| TEXAS INSTRUMENTS INCORPORATED
| Standard Linear and Logic Group
| IBIS Model of SN74CB3T16211
| 3.3-V LOW-VOLTAGE 14-BIT FET BUS SWITCH WITH 5-V-TOLERANT/LEVEL SHIFTER
| This file contains package information for the following:
|  VFBGA 56-pin (GQL) package as [Component] CB3T16211_GQL
|  TSSOP 56-pin (DGG) package as [Component] CB3T16211_DGG
|  TVSOP 56-pin (DGV) package as [Component] CB3T16211_DGV
|  SSOP 56-pin (DL) package as [Component] CB3T16211_DL
| This device can be powered at the following Vccs:
|  3.3 volt Vcc
|  2.5 volt Vcc
| This file provides unique models under the [Model Selector] for each Vcc.
| For operation at a specific Vcc, select the appropriate model after each
| [Model Selector] keyword.
[IBIS Ver]   3.2
[Comment char]  |_char
[File Name]   sn74cb3t16211.ibs
[File Rev]   1.3 | a_die
[Date]   March 23, 2006
[Source]   Data created from TI-SPICE simulations at TI-SLL.
[Notes]   The following is an IBIS list for the CB3T16211.
   Please contact sllibis@ti.com with questions and
   comments concerning SLL IBIS models.
   - FILE REV HISTORY
   - 1.3 Added GQL package information on 03/23/06
   - Non-monotonic data due to FET characteristics.
   - Power clamp data deleted as there is no power-clamp diode.
[Disclaimer] Property of Texas Instruments Incorporated.  Unauthorized
   reproduction and/or distribution is strictly prohibited.
   This product is protected under copyright law.
   Created  2003, (C) Copyright  2003, Texas Instruments
   Incorporated, All Rights Reserved
   UNLESS THERE IS A SIGNED, WRITTEN AGREEMENT TO THE
   CONTRARY, TEXAS INSTRUMENTS (TI) IS PROVIDING THE IBIS
   MODELS  AND WITHOUT ANY WARRANTY, EXPRESSED OR
   IMPLIED.  TI assumes no liability for:
   1) the accuracy of the IBIS models provided to your
   company;
   2) the proper functioning of these IBIS Models in your
   design or for any resulting applications; or
   3) infringement of patents, copyrights or intellectual
   property rights resulting from your use of these IBIS
   models.
   TI provides IBIS Models as a service to our customers.
   You and your company shall not distribute, sell or give
   these models to anyone else without prior written
   permission from TI.
   TI reserves the right to make changes to our products or
   to discontinue any semiconductor product or service
   without notice, and advises our customers to obtain the
   latest version of relevant information to verify, before
   placing orders, that the information being relied on is
   current.
   Please be aware that your receipt and use of the IBIS
   information provided shall serve as acceptance of these
   terms and conditions.  If you do not accept these terms,
   you should return or destroy the IBIS models and any
   other accompanying information immediately.
| Component CB3T16211_GQL 56-pin VFBGA
[Component]   CB3T16211_GQL
[Manufacturer]   Texas Instruments, Inc.
[Package]
|   typ   min   max
R_pkg   6.500e-02   3.500e-02   9.700e-02
L_pkg   1.952e-09   1.000e-09   3.191e-09
C_pkg   2.830e-13   1.620e-13   4.340e-13
[Pin]   signal_name   model_name   R_pin   L_pin   C_pin
A3   NC   NC   3.600e-02   1.004e-09   1.760e-13
A2   1A1   CB3T16211_IO   4.000e-02   1.191e-09   1.860e-13
A1   1A2   CB3T16211_IO   4.700e-02   1.411e-09   2.090e-13
B3   1A3   CB3T16211_IO   9.700e-02   3.191e-09   4.340e-13
B2   1A4   CB3T16211_IO   7.400e-02   2.213e-09   3.290e-13
B1   1A5   CB3T16211_IO   6.000e-02   1.712e-09   2.430e-13
C3   1A6   CB3T16211_IO   8.500e-02   2.691e-09   3.680e-13
C2   GND   GND   7.400e-02   2.160e-09   3.150e-13
C1   1A7   CB3T16211_IO   6.000e-02   1.666e-09   2.470e-13
D2   1A8   CB3T16211_IO   7.400e-02   2.121e-09   3.130e-13
D3   1A9   CB3T16211_IO   9.100e-02   2.924e-09   3.970e-13
D1   1A10   CB3T16211_IO   6.000e-02   1.619e-09   2.450e-13
E2   1A11   CB3T16211_IO   6.900e-02   2.031e-09   2.880e-13
E1   1A12   CB3T16211_IO   6.000e-02   1.583e-09   2.200e-13
F1   2A1   CB3T16211_IO   6.000e-02   1.578e-09   2.200e-13
F2   2A2   CB3T16211_IO   6.900e-02   2.017e-09   2.860e-13
G1   VCC   POWER   6.000e-02   1.594e-09   2.410e-13
G3   2A3   CB3T16211_IO   9.200e-02   2.917e-09   3.970e-13
G2   GND   GND   7.500e-02   2.114e-09   3.150e-13
H1   2A4   CB3T16211_IO   6.000e-02   1.632e-09   2.470e-13
H2   2A5   CB3T16211_IO   7.000e-02   2.074e-09   3.070e-13
H3   2A6   CB3T16211_IO   8.600e-02   2.664e-09   3.650e-13
J1   2A7   CB3T16211_IO   6.000e-02   1.689e-09   2.490e-13
J2   2A8   CB3T16211_IO   6.600e-02   2.152e-09   3.320e-13
J3   2A9   CB3T16211_IO   8.700e-02   3.118e-09   4.230e-13
K1   2A10   CB3T16211_IO   3.800e-02   1.303e-09   2.000e-13
K2   2A11   CB3T16211_IO   3.500e-02   1.176e-09   1.830e-13
K3   2A12   CB3T16211_IO   3.500e-02   1.007e-09   1.620e-13
K4   2B12   CB3T16211_IO   3.500e-02   1.000e-09   1.620e-13
K5   2B11   CB3T16211_IO   3.500e-02   1.154e-09   1.800e-13
K6   2B10   CB3T16211_IO   4.100e-02   1.352e-09   2.040e-13
J4   2B9   CB3T16211_IO   8.800e-02   3.137e-09   4.300e-13
J5   2B8   CB3T16211_IO   7.400e-02   2.218e-09   3.340e-13
J6   2B7   CB3T16211_IO   6.000e-02   1.683e-09   2.500e-13
H4   2B6   CB3T16211_IO   8.500e-02   2.658e-09   3.720e-13
H5   2B5   CB3T16211_IO   7.500e-02   2.149e-09   3.210e-13
H6   2B4   CB3T16211_IO   6.000e-02   1.627e-09   2.480e-13
G5   GND   GND   7.500e-02   2.113e-09   3.140e-13
G4   2B3   CB3T16211_IO   9.200e-02   2.922e-09   3.960e-13
G6   2B2   CB3T16211_IO   6.000e-02   1.594e-09   2.420e-13
F5   2B1   CB3T16211_IO   6.900e-02   2.016e-09   2.880e-13
F6   1B12   CB3T16211_IO   6.000e-02   1.580e-09   2.210e-13
E6   1B11   CB3T16211_IO   6.000e-02   1.582e-09   2.200e-13
E5   1B10   CB3T16211_IO   6.900e-02   2.026e-09   2.890e-13
D6   1B9   CB3T16211_IO   6.000e-02   1.610e-09   2.450e-13
D4   1B8   CB3T16211_IO   9.200e-02   2.933e-09   3.960e-13
D5   1B7   CB3T16211_IO   7.500e-02   2.126e-09   3.110e-13
C6   1B6   CB3T16211_IO   6.000e-02   1.641e-09   2.450e-13
C5   GND   GND   7.300e-02   2.168e-09   3.190e-13
C4   1B5   CB3T16211_IO   8.600e-02   2.675e-09   3.620e-13
B6   1B4   CB3T16211_IO   6.000e-02   1.688e-09   2.430e-13
B5   1B3   CB3T16211_IO   7.500e-02   2.281e-09   3.330e-13
B4   1B2   CB3T16211_IO   9.500e-02   3.168e-09   4.240e-12
A6   1B1   CB3T16211_IO   4.500e-02   1.418e-09   2.090e-12
A5   NOE2   CB3T16211_IN   3.900e-02   1.216e-09   1.900e-12
A4   NOE1   CB3T16211_IN   3.700e-02   1.029e-09   1.790e-12
| Component CB3T16211_DGG 56-pin TSSOP
[Component]   CB3T16211_DGG
[Manufacturer]   Texas Instruments, Inc.
[Package]
|   typ   min   max
R_pkg   4.500e-02   3.500e-02   6.200e-02
L_pkg   3.324e-09   2.403e-09   5.094e-09
C_pkg   5.640e-13   3.410e-13   9.140e-13
[Pin]   signal_name   model_name   R_pin   L_pin   C_pin
1   NC   NC   6.200e-02   5.094e-09   8.560e-13
2   1A1   CB3T16211_IO   6.100e-02   4.621e-09   9.020e-13
3   1A2   CB3T16211_IO   6.000e-02   4.316e-09   8.020e-13
4   1A3   CB3T16211_IO   5.900e-02   3.968e-09   6.980e-13
5   1A4   CB3T16211_IO   5.700e-02   3.716e-09   6.490e-13
6   1A5   CB3T16211_IO   4.200e-02   3.517e-09   6.530e-13
7   1A6   CB3T16211_IO   4.100e-02   3.160e-09   5.700e-13
8   GND   GND   3.900e-02   2.981e-09   4.820e-13
9   1A7   CB3T16211_IO   3.900e-02   2.808e-09   4.470e-13
10   1A8   CB3T16211_IO   3.800e-02   2.715e-09   4.090e-13
11   1A9   CB3T16211_IO   4.100e-02   2.675e-09   3.910e-13
12   1A10   CB3T16211_IO   3.900e-02   2.536e-09   3.660e-13
13   1A11   CB3T16211_IO   3.900e-02   2.457e-09   3.480e-13
14   1A12   CB3T16211_IO   3.800e-02   2.411e-09   3.530e-13
15   2A1   CB3T16211_IO   3.900e-02   2.456e-09   3.550e-13
16   2A2   CB3T16211_IO   3.900e-02   2.471e-09   3.490e-13
17   VCC   POWER   4.000e-02   2.580e-09   3.700e-13
18   2A3   CB3T16211_IO   3.800e-02   2.651e-09   3.890e-13
19   GND   GND   3.800e-02   2.739e-09   4.110e-13
20   2A4   CB3T16211_IO   3.900e-02   2.838e-09   4.490e-13
21   2A5   CB3T16211_IO   3.800e-02   2.988e-09   4.840e-13
22   2A6   CB3T16211_IO   3.800e-02   3.104e-09   5.640e-13
23   2A7   CB3T16211_IO   4.000e-02   3.427e-09   6.380e-13
24   2A8   CB3T16211_IO   5.600e-02   3.654e-09   6.410e-13
25   2A9   CB3T16211_IO   5.700e-02   3.932e-09   7.000e-13
26   2A10   CB3T16211_IO   5.800e-02   4.257e-09   8.060e-13
27   2A11   CB3T16211_IO   5.700e-02   4.580e-09   9.140e-13
28   2A12   CB3T16211_IO   5.900e-02   5.038e-09   8.610e-13
29   2B12   CB3T16211_IO   6.000e-02   5.058e-09   8.580e-13
30   2B11   CB3T16211_IO   5.600e-02   4.543e-09   9.040e-13
31   2B10   CB3T16211_IO   5.700e-02   4.241e-09   8.020e-13
32   2B9   CB3T16211_IO   5.900e-02   3.933e-09   6.990e-13
33   2B8   CB3T16211_IO   5.600e-02   3.616e-09   6.370e-13
34   2B7   CB3T16211_IO   3.700e-02   3.368e-09   6.400e-13
35   2B6   CB3T16211_IO   3.600e-02   3.024e-09   5.630e-13
36   2B5   CB3T16211_IO   3.500e-02   2.876e-09   4.740e-13
37   2B4   CB3T16211_IO   3.500e-02   2.745e-09   4.440e-13
38   GND   GND   3.700e-02   2.683e-09   4.050e-13
39   2B3   CB3T16211_IO   3.800e-02   2.603e-09   3.820e-13
40   2B2   CB3T16211_IO   3.800e-02   2.510e-09   3.620e-13
41   2B1   CB3T16211_IO   3.600e-02   2.412e-09   3.410e-13
42   1B12   CB3T16211_IO   3.800e-02   2.416e-09   3.490e-13
43   1B11   CB3T16211_IO   3.800e-02   2.403e-09   3.490e-13
44   1B10   CB3T16211_IO   3.700e-02   2.429e-09   3.410e-13
45   1B9   CB3T16211_IO   3.600e-02   2.483e-09   3.580e-13
46   1B8   CB3T16211_IO   3.700e-02   2.614e-09   3.810e-13
47   1B7   CB3T16211_IO   3.500e-02   2.669e-09   4.020e-13
48   1B6   CB3T16211_IO   3.600e-02   2.763e-09   4.420e-13
49   GND   GND   3.600e-02   2.942e-09   4.780e-13
50   1B5   CB3T16211_IO   3.500e-02   3.053e-09   5.640e-13
51   1B4   CB3T16211_IO   3.600e-02   3.408e-09   6.410e-13
52   1B3   CB3T16211_IO   5.800e-02   3.698e-09   6.410e-13
53   1B2   CB3T16211_IO   5.900e-02   3.974e-09   6.970e-13
54   1B1   CB3T16211_IO   6.100e-02   4.327e-09   8.020e-13
55   NOE2   CB3T16211_IN   6.100e-02   4.624e-09   9.050e-13
56   NOE1   CB3T16211_IN   6.000e-02   5.063e-09   8.580e-13
| Component CB3T16211_DGV 56-pin TVSOP
[Component]   CB3T16211_DGV
[Manufacturer]   Texas Instruments, Inc.
[Package]
|   typ   min   max
R_pkg   6.300e-02   5.000e-02   8.400e-02
L_pkg   2.945e-09   2.394e-09   3.939e-09
C_pkg   3.910e-13   2.710e-13   5.880e-13
[Pin]   signal_name   model_name   R_pin   L_pin   C_pin
1   NC   NC   6.800e-02   3.933e-09   5.880e-13
2   1A1   CB3T16211_IO   6.800e-02   3.568e-09   5.870e-13
3   1A2   CB3T16211_IO   7.600e-02   3.464e-09   5.150e-13
4   1A3   CB3T16211_IO   8.400e-02   3.444e-09   4.590e-13
5   1A4   CB3T16211_IO   8.100e-02   3.277e-09   4.270e-13
6   1A5   CB3T16211_IO   7.400e-02   3.136e-09   3.870e-13
7   1A6   CB3T16211_IO   6.900e-02   2.970e-09   4.010e-13
8   GND   GND   5.000e-02   2.785e-09   3.790e-13
9   1A7   CB3T16211_IO   5.100e-02   2.685e-09   3.200e-13
10   1A8   CB3T16211_IO   5.300e-02   2.611e-09   3.160e-13
11   1A9   CB3T16211_IO   5.300e-02   2.495e-09   2.970e-13
12   1A10   CB3T16211_IO   5.300e-02   2.435e-09   2.920e-13
13   1A11   CB3T16211_IO   5.500e-02   2.412e-09   2.850e-13
14   1A12   CB3T16211_IO   5.600e-02   2.401e-09   2.730e-13
15   2A1   CB3T16211_IO   5.500e-02   2.401e-09   2.730e-13
16   2A2   CB3T16211_IO   5.500e-02   2.399e-09   2.840e-13
17   VCC   POWER   5.400e-02   2.406e-09   2.890e-13
18   2A3   CB3T16211_IO   5.300e-02   2.450e-09   2.930e-13
19   GND   GND   5.100e-02   2.544e-09   3.110e-13
20   2A4   CB3T16211_IO   5.100e-02   2.626e-09   3.150e-13
21   2A5   CB3T16211_IO   5.000e-02   2.727e-09   3.690e-13
22   2A6   CB3T16211_IO   6.500e-02   2.903e-09   3.930e-13
23   2A7   CB3T16211_IO   7.500e-02   3.091e-09   3.860e-13
24   2A8   CB3T16211_IO   8.200e-02   3.272e-09   4.280e-13
25   2A9   CB3T16211_IO   8.200e-02   3.393e-09   4.570e-13
26   2A10   CB3T16211_IO   7.300e-02   3.380e-09   5.080e-13
27   2A11   CB3T16211_IO   7.100e-02   3.577e-09   5.800e-13
28   2A12   CB3T16211_IO   6.800e-02   3.937e-09   5.740e-13
29   2B12   CB3T16211_IO   6.900e-02   3.923e-09   5.690e-13
30   2B11   CB3T16211_IO   6.400e-02   3.536e-09   5.740e-13
31   2B10   CB3T16211_IO   7.600e-02   3.428e-09   5.170e-13
32   2B9   CB3T16211_IO   8.100e-02   3.395e-09   4.680e-13
33   2B8   CB3T16211_IO   8.000e-02   3.255e-09   4.310e-13
34   2B7   CB3T16211_IO   7.100e-02   3.064e-09   3.860e-13
35   2B6   CB3T16211_IO   6.100e-02   2.878e-09   3.890e-13
36   2B5   CB3T16211_IO   5.000e-02   2.710e-09   3.630e-13
37   2B4   CB3T16211_IO   5.000e-02   2.606e-09   3.110e-13
38   GND   GND   5.200e-02   2.534e-09   3.060e-13
39   2B3   CB3T16211_IO   5.200e-02   2.439e-09   2.890e-13
40   2B2   CB3T16211_IO   5.300e-02   2.399e-09   2.860e-13
41   2B1   CB3T16211_IO   5.500e-02   2.394e-09   2.820e-13
42   1B12   CB3T16211_IO   5.500e-02   2.398e-09   2.710e-13
43   1B11   CB3T16211_IO   5.600e-02   2.396e-09   2.710e-13
44   1B10   CB3T16211_IO   5.400e-02   2.402e-09   2.830e-13
45   1B9   CB3T16211_IO   5.400e-02   2.423e-09   2.880e-13
46   1B8   CB3T16211_IO   5.300e-02   2.474e-09   2.920e-13
47   1B7   CB3T16211_IO   5.100e-02   2.569e-09   3.090e-13
48   1B6   CB3T16211_IO   5.100e-02   2.638e-09   3.130e-13
49   GND   GND   5.100e-02   2.742e-09   3.660e-13
50   1B5   CB3T16211_IO   6.400e-02   2.917e-09   3.900e-13
51   1B4   CB3T16211_IO   7.400e-02   3.083e-09   3.830e-13
52   1B3   CB3T16211_IO   8.100e-02   3.249e-09   4.300e-13
53   1B2   CB3T16211_IO   8.300e-02   3.400e-09   4.550e-13
54   1B1   CB3T16211_IO   7.500e-02   3.427e-09   5.050e-13
55   NOE2   CB3T16211_IN   7.100e-02   3.585e-09   5.780e-13
56   NOE1   CB3T16211_IN   6.900e-02   3.939e-09   5.810e-13
| Component CB3T16211_DL 56-pin SSOP
[Component]   CB3T16211_DL
[Manufacturer]   Texas Instruments, Inc.
[Package]
|   typ   min   max
R_pkg   5.500e-02   4.800e-02   6.700e-02
L_pkg   6.539e-09   4.803e-09   9.746e-09
C_pkg   8.570e-13   5.000e-13   1.351e-12
[Pin]   signal_name   model_name   R_pin   L_pin   C_pin
1   NC   NC   6.400e-02   9.646e-09   1.202e-12
2   1A1   CB3T16211_IO   5.900e-02   8.723e-09   1.348e-12
3   1A2   CB3T16211_IO   5.900e-02   8.139e-09   1.223e-12
4   1A3   CB3T16211_IO   5.600e-02   7.554e-09   1.088e-12
5   1A4   CB3T16211_IO   5.400e-02   6.991e-09   9.660e-13
6   1A5   CB3T16211_IO   5.300e-02   6.659e-09   9.730e-13
7   1A6   CB3T16211_IO   5.500e-02   6.321e-09   9.050e-13
8   GND   GND   5.600e-02   5.942e-09   7.130e-13
9   1A7   CB3T16211_IO   5.700e-02   5.768e-09   6.780e-13
10   1A8   CB3T16211_IO   5.400e-02   5.459e-09   6.310e-13
11   1A9   CB3T16211_IO   5.100e-02   5.224e-09   6.380e-13
12   1A10   CB3T16211_IO   4.800e-02   5.088e-09   6.010e-13
13   1A11   CB3T16211_IO   5.000e-02   5.021e-09   5.180e-13
14   1A12   CB3T16211_IO   5.100e-02   4.803e-09   5.000e-13
15   2A1   CB3T16211_IO   5.100e-02   4.803e-09   5.000e-13
16   2A2   CB3T16211_IO   5.000e-02   5.021e-09   5.180e-13
17   VCC   POWER   4.800e-02   5.088e-09   6.010e-13
18   2A3   CB3T16211_IO   5.100e-02   5.224e-09   6.380e-13
19   GND   GND   5.400e-02   5.459e-09   6.310e-13
20   2A4   CB3T16211_IO   5.700e-02   5.768e-09   6.770e-13
21   2A5   CB3T16211_IO   5.500e-02   5.942e-09   7.150e-13
22   2A6   CB3T16211_IO   5.500e-02   6.321e-09   9.070e-13
23   2A7   CB3T16211_IO   5.300e-02   6.659e-09   9.720e-13
24   2A8   CB3T16211_IO   5.400e-02   6.991e-09   9.660e-13
25   2A9   CB3T16211_IO   5.600e-02   7.554e-09   1.087e-12
26   2A10   CB3T16211_IO   5.900e-02   8.139e-09   1.223e-12
27   2A11   CB3T16211_IO   5.900e-02   8.727e-09   1.351e-12
28   2A12   CB3T16211_IO   6.700e-02   9.746e-09   1.210e-12
29   2B12   CB3T16211_IO   6.300e-02   9.630e-09   1.203e-12
30   2B11   CB3T16211_IO   6.000e-02   8.751e-09   1.349e-12
31   2B10   CB3T16211_IO   6.000e-02   8.184e-09   1.224e-12
32   2B9   CB3T16211_IO   5.600e-02   7.543e-09   1.087e-12
33   2B8   CB3T16211_IO   5.400e-02   7.005e-09   9.690e-13
34   2B7   CB3T16211_IO   5.600e-02   6.714e-09   9.750e-13
35   2B6   CB3T16211_IO   5.800e-02   6.384e-09   9.090e-13
36   2B5   CB3T16211_IO   5.700e-02   5.976e-09   7.170e-13
37   2B4   CB3T16211_IO   5.700e-02   5.743e-09   6.770e-13
38   GND   GND   5.400e-02   5.468e-09   6.310e-13
39   2B3   CB3T16211_IO   5.500e-02   5.329e-09   6.440e-13
40   2B2   CB3T16211_IO   5.200e-02   5.189e-09   6.060e-13
41   2B1   CB3T16211_IO   5.200e-02   5.053e-09   5.190e-13
42   1B12   CB3T16211_IO   5.200e-02   4.825e-09   5.020e-13
43   1B11   CB3T16211_IO   5.400e-02   4.897e-09   5.060e-13
44   1B10   CB3T16211_IO   5.200e-02   5.093e-09   5.210e-13
45   1B9   CB3T16211_IO   5.100e-02   5.179e-09   6.080e-13
46   1B8   CB3T16211_IO   5.400e-02   5.314e-09   6.450e-13
47   1B7   CB3T16211_IO   5.500e-02   5.511e-09   6.320e-13
48   1B6   CB3T16211_IO   5.700e-02   5.770e-09   6.770e-13
49   GND   GND   5.600e-02   5.956e-09   7.160e-13
50   1B5   CB3T16211_IO   5.500e-02   6.320e-09   9.050e-13
51   1B4   CB3T16211_IO   5.200e-02   6.621e-09   9.680e-13
52   1B3   CB3T16211_IO   5.300e-02   6.974e-09   9.660e-13
53   1B2   CB3T16211_IO   5.700e-02   7.571e-09   1.089e-12
54   1B1   CB3T16211_IO   5.700e-02   8.097e-09   1.219e-12
55   NOE2   CB3T16211_IN   5.900e-02   8.723e-09   1.349e-12
56   NOE1   CB3T16211_IN   6.100e-02   9.560e-09   1.199e-12
[Series Switch Groups]
| Function Group States
On  1 /   | 1A1-1A12->1B1-1B12 NOE1 LOW
On  2 /   | 2A1-2A12->2B1-2B12 NOE2 LOW
On  1 2  /   | Enable Both
Off 1 /   | 1A1-1A12->1B1-1B12 NOE1 HIGH
Off 2 /   | 2A1-2A12->2B1-2B12 NOE2 HIGH
Off 1 2 /   | Disable Both
[Series Pin Mapping]   pin_2   model_name   function_table_group
2   54   CB3T16211_IO_33_S   1
| 2   54   CB3T16211_IO_25_S   1
3   53   CB3T16211_IO_33_S   1
| 3   53   CB3T16211_IO_25_S   1
4   52   CB3T16211_IO_33_S   1
| 4   52   CB3T16211_IO_25_S   1
5   51   CB3T16211_IO_33_S   1
| 5   51   CB3T16211_IO_25_S   1
6   50   CB3T16211_IO_33_S   1
| 6   50   CB3T16211_IO_25_S   1
7   48   CB3T16211_IO_33_S   1
| 7   48   CB3T16211_IO_25_S   1
9   47   CB3T16211_IO_33_S   1
| 9   47   CB3T16211_IO_25_S   1
10   46   CB3T16211_IO_33_S   1
| 10   46   CB3T16211_IO_25_S   1
11   45   CB3T16211_IO_33_S   1
| 11   45   CB3T16211_IO_25_S   1
12   44   CB3T16211_IO_33_S   1
| 12   44   CB3T16211_IO_25_S   1
13   43   CB3T16211_IO_33_S   1
| 13   43   CB3T16211_IO_25_S   1
14   42   CB3T16211_IO_33_S   1
| 14   42   CB3T16211_IO_25_S   1
15   41   CB3T16211_IO_33_S   2
| 15   41   CB3T16211_IO_25_S   2
16   40   CB3T16211_IO_33_S   2
| 16   40   CB3T16211_IO_25_S   2
18   39   CB3T16211_IO_33_S   2
| 18   39   CB3T16211_IO_25_S   2
20   37   CB3T16211_IO_33_S   2
| 20   37   CB3T16211_IO_25_S   2
21   36   CB3T16211_IO_33_S   2
| 21   36   CB3T16211_IO_25_S   2
22   35   CB3T16211_IO_33_S   2
| 22   35   CB3T16211_IO_25_S   2
23   34   CB3T16211_IO_33_S   2
| 23   34   CB3T16211_IO_25_S   2
24   33   CB3T16211_IO_33_S   2
| 24   33   CB3T16211_IO_25_S   2
25   32   CB3T16211_IO_33_S   2
| 25   32   CB3T16211_IO_25_S   2
26   31   CB3T16211_IO_33_S   2
| 26   31   CB3T16211_IO_25_S   2
27   30   CB3T16211_IO_33_S   2
| 27   30   CB3T16211_IO_25_S   2
28   29   CB3T16211_IO_33_S   2
| 28   29   CB3T16211_IO_25_S   2
| Model CB3T16211_IN
[Model Selector]   CB3T16211_IN
CB3T16211_IN_33   3.3 volt Vcc
CB3T16211_IN_25   2.5 volt Vcc
| Model CB3T16211_IO
[Model Selector]   CB3T16211_IO
CB3T16211_IO_33   3.3 volt Vcc
CB3T16211_IO_25   2.5 volt Vcc
| Model CB3T16211_IO_S
[Model Selector]   CB3T16211_IO_S
CB3T16211_IO_33_S   3.3 volt Vcc
CB3T16211_IO_25_S   2.5 volt Vcc
[Model]   CB3T16211_IO_33_S
Model_type  Series_switch
| variable   typ   min   max
C_comp   0   0   0
[Temperature Range]   40   100   -40
| Ambient temperature   25   85   -40
[Voltage range]   3.3   3   3.6
[On]
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[Off]
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[Model]   CB3T16211_IO_25_S
Model_type  Series_switch
| variable   typ   min   max
C_comp   0   0   0
[Temperature Range]   40   100   -40
| Ambient temperature   25   85   -40
[Voltage range]   2.5   2.3   2.7
[On]
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[Off]
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| Models and submodels in the file (6): CB3T16211_IN_33 (Input), CB3T16211_IN_25 (Input), CB3T16211_IO_33_S (Series_switch), CB3T16211_IO_33 (Terminator), CB3T16211_IO_25_S (Series_switch), CB3T16211_IO_25 (Terminator)
